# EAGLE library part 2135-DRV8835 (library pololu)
https://www.pololu.com/product/2135 This tiny breakout board for TI’s DRV8835 dual motor driver can deliver 1.2 A per channel continuously (1.5 A peak) to a pair of DC motors, and it supports two possible control interfaces for added flexibility of use: IN/IN and PHASE/ENABLE. With an operating voltage range from 0 V to 11 V and built-in protection against reverse-voltage, under-voltage, over-current, and over-temperature, this driver is a great solution for powering up to two small, low-voltage motors. The carrier board has the form factor of a 14-pin DIP package, which makes it easy to use with standard solderless breadboards and 0.1″ perfboards.
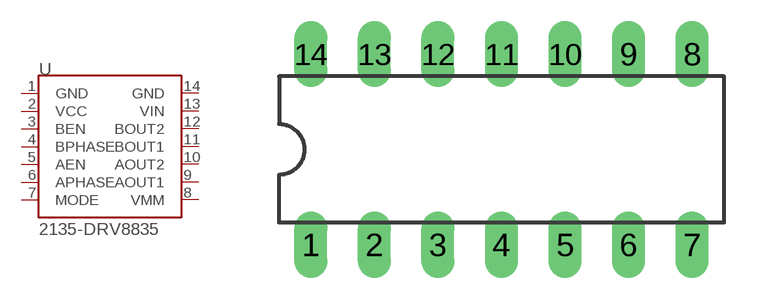
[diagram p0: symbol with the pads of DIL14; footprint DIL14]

Designator prefix U

## 2135-DRV8835  [DIL14]
1  GND  pwr
2  VCC  pwr
3  BEN  in
4  BPHASE  in
5  AEN  in
6  APHASE  in
7  MODE  in
8  VMM  out
9  AOUT1  out
10  AOUT2  out
11  BOUT1  out
12  BOUT2  out
13  VIN  pwr
14  GND  pwr

## Footprint DIL14 (pad centres in mm)
Dual In Line Package
drill 0.813 long: 1 -7.62,-3.81; 2 -5.08,-3.81; 3 -2.54,-3.81; 4 0,-3.81; 5 2.54,-3.81; 6 5.08,-3.81; 7 7.62,-3.81; 8 7.62,3.81; 9 5.08,3.81; 10 2.54,3.81; 11 0,3.81; 12 -2.54,3.81; 13 -5.08,3.81; 14 -7.62,3.81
